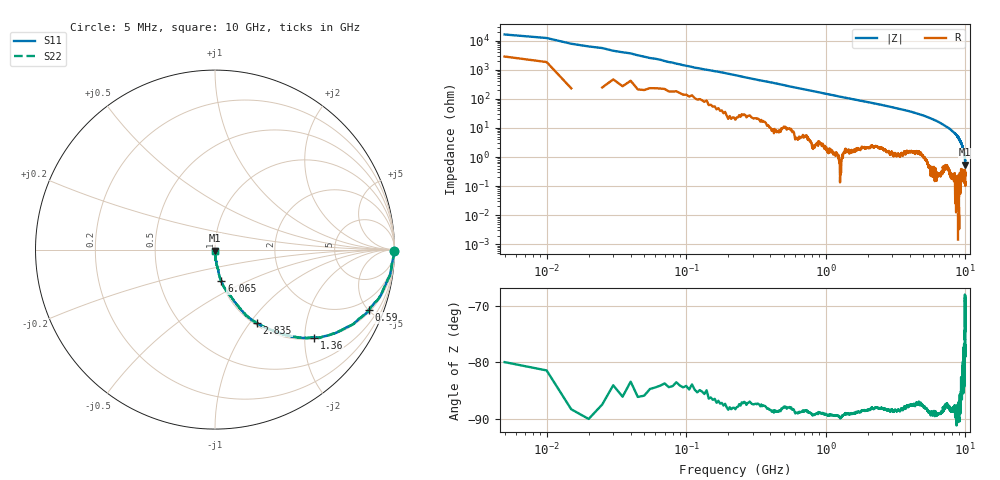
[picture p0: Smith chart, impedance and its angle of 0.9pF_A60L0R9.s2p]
! Amotech Co.,Ltd.
! http://www.amotech.co.kr/
! Part Number: A60L0R9
! These Parameters are Measured in Series Mode Connection
! Operation Temp=25[degC], DC Bias Voltage=0[V]
! Freq. Start=5[MHz] Stop=10[GHz], 2000[Steps]
! Date: Monday, July 14, 2020, 09:26:58
# GHZ S RI R 50.000000
!Freq.(Hz) S11(Real) S11(Imag) S21(Real) S21(Imag) S12(Real) S12(Imag) S22(Real) S22(Imag)
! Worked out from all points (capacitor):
!   2000 points, 5 MHz to 10 GHz, reference 50 ohm
!   read as one part in series: C = 1.15 pF near 55 MHz
!   lowest |Z| = 538 mohm at 9.995 GHz (marker M1)
!   S11 on the Smith chart (normalised r, x): 5 MHz: open; 590 MHz: 1.14, -5.02; 1.36 GHz: 1.03, -2.22; 2.835 GHz: 1.03, -1.09; 6.065 GHz: 1.01, -0.37; 10 GHz: 1.00, -0.01
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0.005  0.9989 -0.00602  0.0011 0.00602  0.0011 0.00602  0.9989 -0.00602
0.065  0.9934 -0.0443  0.00656 0.0443  0.00656 0.0443  0.9934 -0.0443
0.08  0.9911 -0.0558  0.00887 0.0558  0.00887 0.0558  0.9911 -0.0558
0.115  0.9856 -0.0824  0.0144 0.0824  0.0144 0.0824  0.9856 -0.0824
0.16  0.9809 -0.1093  0.0191 0.1093  0.0191 0.1093  0.9809 -0.1093
0.245  0.966 -0.1619  0.034 0.1619  0.034 0.1619  0.966 -0.1619
0.325  0.9435 -0.2083  0.0565 0.2083  0.0565 0.2083  0.9435 -0.2083
0.59  0.8563 -0.3369  0.1437 0.3369  0.1437 0.3369  0.8563 -0.3369
0.95  0.7082 -0.4455  0.2918 0.4455  0.2918 0.4455  0.7082 -0.4455
1.36  0.5507 -0.4904  0.4493 0.4904  0.4493 0.4904  0.5507 -0.4904
1.675  0.4549 -0.488  0.5451 0.488  0.5451 0.488  0.4549 -0.488
2.835  0.234 -0.4106  0.766 0.4106  0.766 0.4106  0.234 -0.4106
3.34  0.1768 -0.3685  0.8232 0.3685  0.8232 0.3685  0.1768 -0.3685
5.005  0.0738 -0.2435  0.9262 0.2435  0.9262 0.2435  0.0738 -0.2435
6.065  0.0355 -0.1767  0.9645 0.1767  0.9645 0.1767  0.0355 -0.1767
6.67  0.023 -0.1413  0.977 0.1413  0.977 0.1413  0.023 -0.1413
8.335  0.00624 -0.0673  0.9938 0.0673  0.9938 0.0673  0.00624 -0.0673
8.885  0.00312 -0.0495  0.9969 0.0495  0.9969 0.0495  0.00312 -0.0495
9.545  0.0025 -0.0221  0.9975 0.0221  0.9975 0.0221  0.0025 -0.0221
9.875  0.00213 -0.0118  0.9979 0.0118  0.9979 0.0118  0.00213 -0.0118
9.995  0.00105 -0.00528  0.9989 0.00528  0.9989 0.00528  0.00105 -0.00528
10  0.00139 -0.00584  0.9986 0.00584  0.9986 0.00584  0.00139 -0.00584
